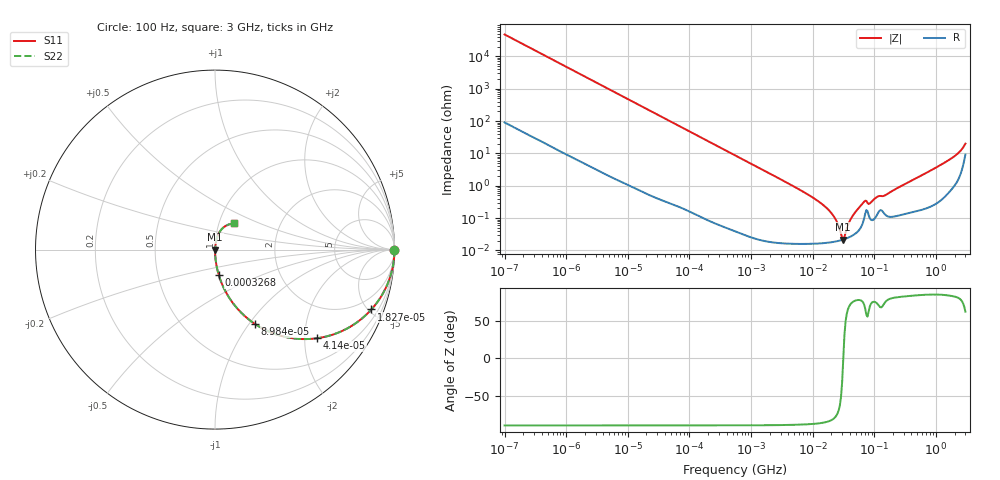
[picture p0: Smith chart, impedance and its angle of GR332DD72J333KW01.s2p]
!Murata Part Number: GR332DD72J333KW01
!These Parameters are Measured in Series Mode Connection
!Data Generated on Jun 10, 2025
!  o--ll--o
!Port1  Port2
!  o------o
!Operation Temp=25[degC], DC Bias Voltage=0[V]
!Freq. Start=100[Hz] Stop=3[GHz] 401[Steps]
# Hz S RI R 50
!Freq.(Hz) S11(Real) S11(Imag) S21(Real) S21(Imag) S12(Real) S12(Imag) S22(Real) S22(Imag)
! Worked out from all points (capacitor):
!   401 points, 100 Hz to 3 GHz, reference 50 ohm
!   read as one part in series: C = 33.6 nF near 109 Hz
!   lowest |Z| = 21.7 mohm at 31.31 MHz (marker M1)
!   series resonance near 31.29 MHz, so ESL is about 770 pH
!   S11 on the Smith chart (normalised r, x): 100 Hz: open; 18.27 kHz: 1.01, -5.22; 41.4 kHz: 1.01, -2.31; 89.84 kHz: 1.00, -1.07; 326.8 kHz: 1.00, -0.29; 3 GHz: 1.18, +0.36
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100  1 -0.00211  8.5e-06 0.00211  8.5e-06 0.00211  1 -0.00211
1788  0.9985 -0.0375  0.00149 0.0375  0.00149 0.0375  0.9985 -0.0375
6504  0.9814 -0.1339  0.0186 0.1339  0.0186 0.1339  0.9814 -0.1339
18274  0.8716 -0.3334  0.1284 0.3334  0.1284 0.3334  0.8716 -0.3334
31977  0.6901 -0.4612  0.3099 0.4612  0.3099 0.4612  0.6901 -0.4612
41399  0.5711 -0.4935  0.4289 0.4935  0.4289 0.4935  0.5711 -0.4935
89839  0.2218 -0.4138  0.7782 0.4138  0.7782 0.4138  0.2218 -0.4138
157206  0.0858 -0.2784  0.9142 0.2784  0.9142 0.2784  0.0858 -0.2784
326774  0.0216 -0.1436  0.9784 0.1436  0.9784 0.1436  0.0216 -0.1436
547723  0.00801 -0.0869  0.992 0.0869  0.992 0.0869  0.00801 -0.0869
9794414  0.000181 -0.00444  0.9998 0.00444  0.9998 0.00444  0.000181 -0.00444
2.035898e7  0.000182 -0.00137  0.9998 0.00137  0.9998 0.00137  0.000182 -0.00137
2.418395e7  0.000192 -0.000807  0.9998 0.000807  0.9998 0.000807  0.000192 -0.000807
2.872754e7  0.000207 -0.000266  0.9998 0.000266  0.9998 0.000266  0.000207 -0.000266
3.131008e7  0.000217 1.6e-06  0.9998 -1.6e-06  0.9998 -1.6e-06  0.000217 1.6e-06
4.418008e7  0.00029 0.00112  0.9997 -0.00112  0.9997 -0.00112  0.00029 0.00112
6.508213e7  0.000722 0.0028  0.9993 -0.0028  0.9993 -0.0028  0.000722 0.0028
8.425944e7  0.000999 0.00266  0.999 -0.00266  0.999 -0.00266  0.000999 0.00266
1.138854e8  0.00142 0.00444  0.9986 -0.00444  0.9986 -0.00444  0.00142 0.00444
1.751444e8  0.00113 0.006  0.9989 -0.006  0.9989 -0.006  0.00113 0.006
1.573002e9  0.00932 0.0592  0.9907 -0.0592  0.9907 -0.0592  0.00932 0.0592
3e9  0.1082 0.1456  0.8918 -0.1456  0.8918 -0.1456  0.1082 0.1456
